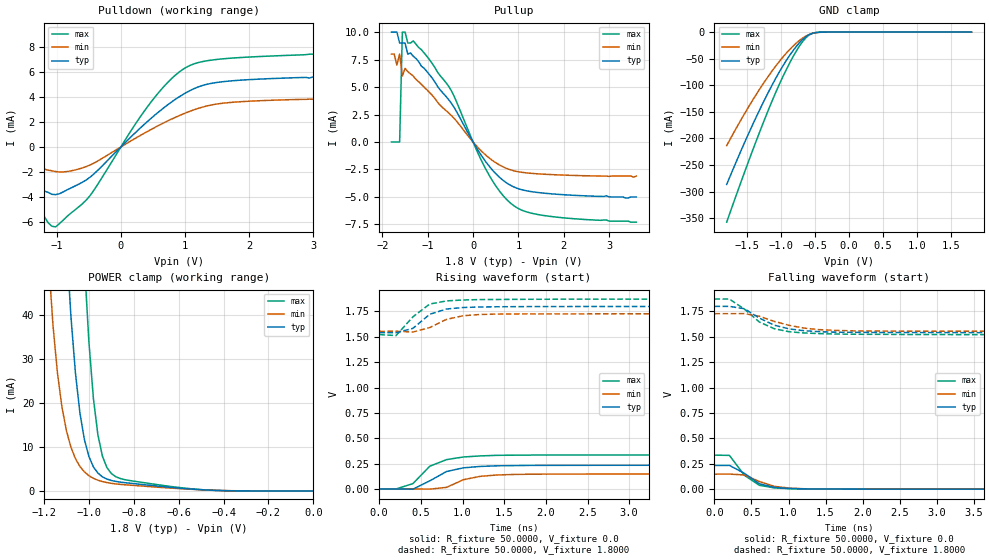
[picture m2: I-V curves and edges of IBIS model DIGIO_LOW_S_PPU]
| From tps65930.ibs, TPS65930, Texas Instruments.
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|   Model DIGIO_LOW_S_PPU
[Model]  DIGIO_LOW_S_PPU
Model_type I/O
Polarity   Non-Inverting
Enable   Active-Low
Vinl =   0.6300V
Vinh =   1.1700V
C_comp   1.0177pF   1.9063pF   1.0043pF
[Temperature Range]   25.0000   0.1250k   -40.0000
[Pullup Reference]   1.8000V   1.7280V   1.8720V
[Pulldown Reference]   0.0V   0.0V   0.0V
[POWER Clamp Reference]   1.8000V   1.7280V   1.8720V
[GND Clamp Reference]   0.0V   0.0V   0.0V
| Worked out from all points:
|   slope of the pulldown table from 0 to 0.27 V, typ, clamps not added: 200 ohm
|   slope of the pullup table from 0 to 0.27 V, typ, clamps not added: 155 ohm
|   GND clamp passes 1 mA (typ) near -0.49 V on its own axis
|   POWER clamp passes 1 mA (typ) near -0.68 V on its own axis
|   rising waveform, R_fixture 50.0000, V_fixture 0.0: 20-80 % time 366ps typ, 328ps min, 320ps max; typ from 0 V to 0.234 V
|   rising waveform, R_fixture 50.0000, V_fixture 1.8000: 20-80 % time 290ps typ, 331ps min, 283ps max; typ from 1.54 V to 1.8 V
|   falling waveform, R_fixture 50.0000, V_fixture 0.0: 20-80 % time 320ps typ, 327ps min, 278ps max; typ from 0.234 V to 0 V
|   falling waveform, R_fixture 50.0000, V_fixture 1.8000: 20-80 % time 462ps typ, 546ps min, 426ps max; typ from 1.8 V to 1.54 V
[Pulldown]
|Voltage   I(typ)   I(min)   I(max)
-1.8V     -600uA     -700uA     -400uA
-1.5V     -2.3mA     -1.2mA     -1.3mA
-1.26V    -3.3mA     -1.66mA    -4.9mA
-1.02V    -3.79mA    -1.95mA    -6.36mA
-480mV    -2.393mA   -1.424mA   -3.854mA
960mV     4.169mA    2.618mA    6.171mA
3.24V     6mA        3.8mA      8mA
3.3V      6mA        4mA        7mA
3.42V     5mA        4mA        8mA
3.48V     6mA        4mA        10mA
3.54V     6mA        4mA        0A
3.6V      10mA       4mA        100mA
[Pullup]
|Voltage   I(typ)   I(min)   I(max)
-1.8V     10mA       8mA        0A
-1.68V    10mA       7mA        0A
-1.62V    9mA        8mA        0A
-1.56V    9mA        6mA        10mA
-1.5V     9mA        6.7mA      10mA
-1.44V    8mA        6.4mA      9mA
-1.32V    7.8mA      6mA        9.2mA
-540mV    3.862mA    2.649mA    5.077mA
300mV     -1.913mA   -1.268mA   -2.623mA
840mV     -3.974mA   -2.553mA   -5.614mA
1.56V     -4.656mA   -2.933mA   -6.691mA
3.6V      -5mA       -3.1mA     -7.3mA
[GND_clamp]
|Voltage   I(typ)   I(min)   I(max)
-1.8V     -286.5mA   -213.6mA   -357.5mA
-1.6V     -226.1mA   -167.3mA   -285.5mA
-1.4V     -169.1mA   -124.3mA   -216.2mA
-1.24V    -126.5mA   -92.77mA   -163.4mA
-1.08V    -87.22mA   -64.16mA   -113.8mA
-920mV    -52.71mA   -39.18mA   -69.69mA
-800mV    -30.79mA   -23.43mA   -40.81mA
-680mV    -13.46mA   -11mA      -17.28mA
-600mV    -5.66mA    -5.217mA   -6.608mA
-520mV    -1.61mA    -1.858mA   -1.531mA
-400mV    -127.8uA   -237.3uA   -89.87uA
1.8V      18.32nA    658.7nA    -876.6nA
[POWER_clamp]
|Voltage   I(typ)   I(min)   I(max)
-1.8V     70.11A     2.031A     796.1A
-1.18V    166.2mA    52.51mA    317.3mA
-1.16V    132.1mA    37.49mA    274.5mA
-1.12V    77.41mA    18.99mA    197.9mA
-1.1V     56.35mA    13.62mA    163mA
-1.08V    39.49mA    9.894mA    130.5mA
-1.06V    26.73mA    7.319mA    100.7mA
-1.02V    11.63mA    4.313mA    51.58mA
-980mV    5.456mA    2.858mA    20.98mA
-940mV    3.208mA    2.125mA    7.923mA
-880mV    2.15mA     1.593mA    3.216mA
0V        18.32nA    51.54nA    21.54nA
[Ramp]
| variable   typ   min   max
dV/dt_r  0.1402/0.3627n   88.5000m/0.3250n   0.2009/0.3173n
dV/dt_f  0.1554/0.4574n   0.1044/0.5408n   0.2100/0.4222n
R_load = 50.0000
[Rising Waveform]
R_fixture= 50.0000
V_fixture= 0.0
V_fixture_min= 0.0
V_fixture_max= 0.0
|time   V(typ)   V(min)   V(max)
0s        0V         0V         0V
202ps     213.6uV    20.5uV     308.6uV
404ps     -1.909mV   210uV      52.66mV
606ps     79.77mV    -1.658mV   223.9mV
808ps     172.2mV    16.01mV    289.5mV
1.01ns    208.3mV    91.28mV    315.3mV
1.212ns   222.2mV    124.5mV    325.9mV
1.414ns   228.2mV    137.9mV    331.7mV
2.424ns   233.3mV    147mV      334.7mV
20ns      233.7mV    147.5mV    334.8mV
[Rising Waveform]
R_fixture= 50.0000
V_fixture= 1.8000
V_fixture_min= 1.7280
V_fixture_max= 1.8720
|time   V(typ)   V(min)   V(max)
0s        1.541V     1.554V     1.522V
202ps     1.54V      1.555V     1.512V
404ps     1.583V     1.547V     1.697V
606ps     1.722V     1.591V     1.823V
808ps     1.774V     1.672V     1.854V
1.01ns    1.789V     1.708V     1.863V
1.212ns   1.794V     1.72V      1.867V
1.616ns   1.797V     1.725V     1.869V
2.626ns   1.799V     1.727V     1.871V
20ns      1.8V       1.728V     1.872V
[Falling Waveform]
R_fixture= 50.0000
V_fixture= 0.0
V_fixture_min= 0.0
V_fixture_max= 0.0
|time   V(typ)   V(min)   V(max)
0s        233.7mV    147.5mV    334.8mV
202ps     234mV      148.3mV    332.9mV
404ps     156.2mV    140.3mV    136.9mV
606ps     53.59mV    75.21mV    37.98mV
808ps     17.36mV    27.75mV    12.54mV
1.01ns    6.851mV    10.46mV    4.54mV
1.212ns   2.987mV    3.882mV    1.931mV
1.414ns   1.435mV    1.799mV    890.8uV
2.222ns   173.4uV    384.9uV    45.82uV
20ns      0V         689nV      0V
[Falling Waveform]
R_fixture= 50.0000
V_fixture= 1.8000
V_fixture_min= 1.7280
V_fixture_max= 1.8720
|time   V(typ)   V(min)   V(max)
0s        1.8V       1.728V     1.872V
202ps     1.8V       1.728V     1.872V
404ps     1.777V     1.729V     1.773V
606ps     1.685V     1.703V     1.646V
808ps     1.615V     1.652V     1.58V
1.01ns    1.578V     1.613V     1.55V
1.212ns   1.56V      1.586V     1.538V
1.616ns   1.546V     1.564V     1.528V
4.242ns   1.541V     1.554V     1.522V
20ns      1.541V     1.554V     1.522V
